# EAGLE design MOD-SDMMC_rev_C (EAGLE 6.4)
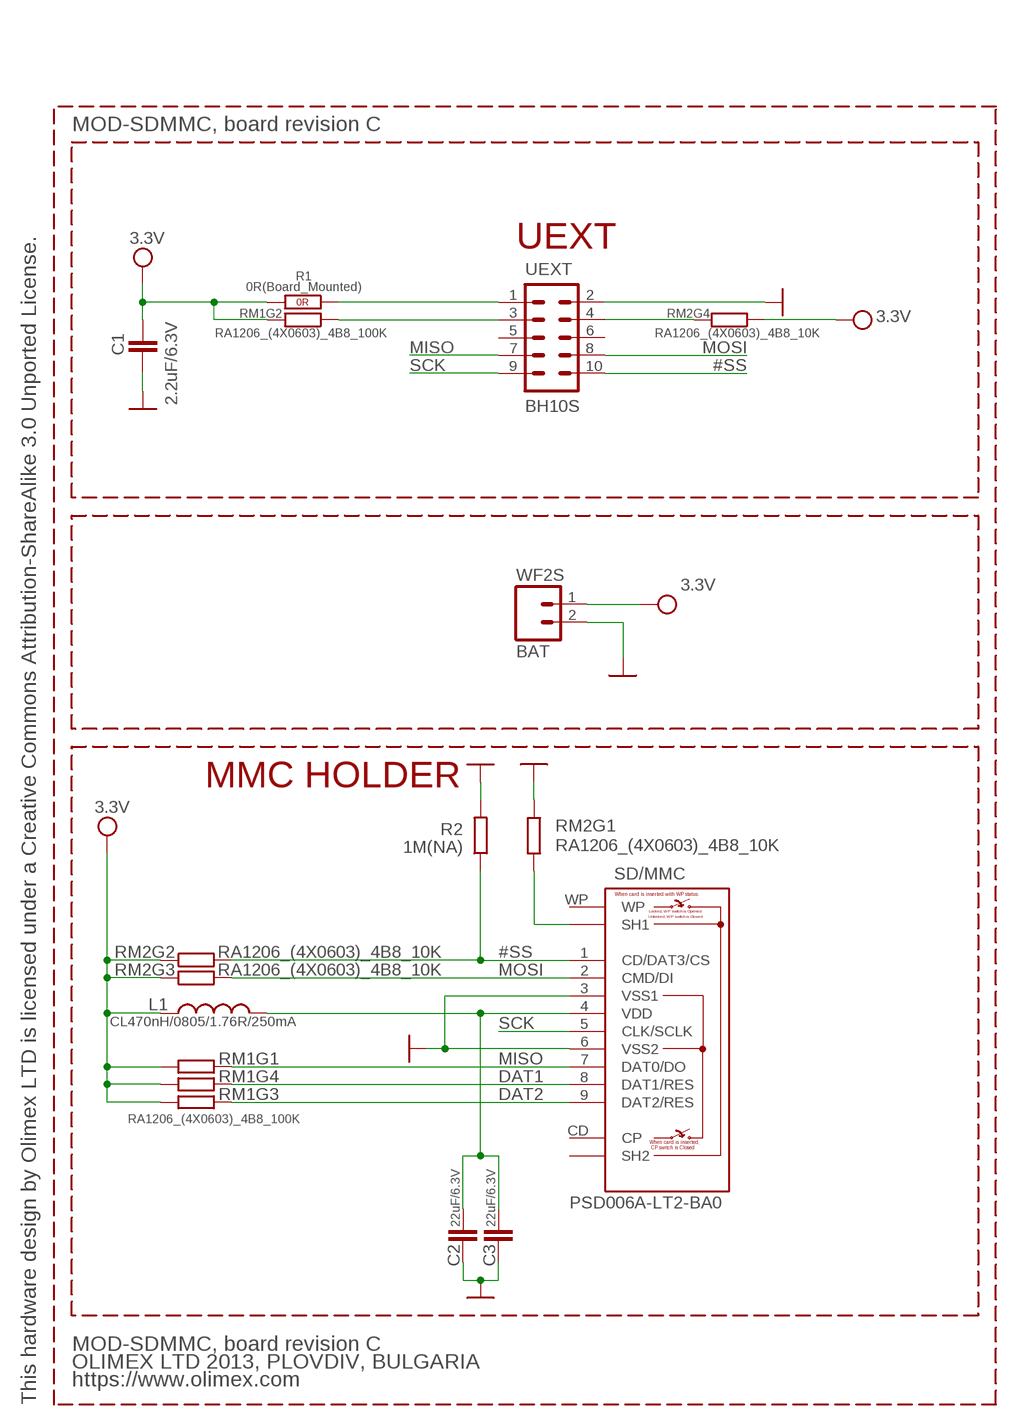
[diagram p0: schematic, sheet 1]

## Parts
BAT  WF2S  CON2PV2-2.54MM  [CON2.54MM-2-0]
C1  2.2uF/6.3V  C-EUC0603_DWS  [C0603_DWS]
C2  22uF/6.3V  C-EUC0603_DWS  [C0603_DWS]
C3  22uF/6.3V  C-EUC0603_DWS  [C0603_DWS]
L1  CL470nH/0805/1.76R/250mA  L-USL0805_5MIL_DWS  [L0805_5MIL_DWS]
R1  0R(Board_Mounted)  R_0R0R(NA)  [0603_0R]
R2  1M(NA)  R-EU_R0603_5MIL_DWS  [R0603_5MIL_DWS]
RM1  RA1206_(4X0603)_4B8_100K  R_MATRIX_4E  [R_MATRIX_4]
RM2  RA1206_(4X0603)_4B8_10K  R_MATRIX_4E  [R_MATRIX_4]
SD/MMC  PSD006A-LT2-BA0  SD_CARD_PSD006A-LT2-BA0  [SD_CARD]
UEXT  BH10S  ML10  [ML10-MALE]

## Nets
#SS: R2.1 RM2.2.2 SD/MMC.1(CD/DAT3/CS) UEXT.10
DAT1: RM1.4.1 SD/MMC.8(DAT1/RES)
DAT2: RM1.3.1 SD/MMC.9(DAT2/RES)
GND: BAT.2 C1.1 C2.1 C3.1 R2.2 RM2.1.1 SD/MMC.3(VSS1) SD/MMC.6(VSS2) UEXT.2
MISO: RM1.1.1 SD/MMC.7(DAT0/DO) UEXT.7
MOSI: RM2.3.2 SD/MMC.2(CMD/DI) UEXT.8
N$1: RM2.1.2 SD/MMC.SH1
N$2: RM1.2.1 UEXT.3
N$3 [PWR]: R1.1(1.1) UEXT.1
N$4: RM2.4.2 UEXT.4
SCK: SD/MMC.5(CLK/SCLK) UEXT.9
VCC [PWR]: BAT.1 C1.2 L1.1 R1.2(1.2) RM1.1.2 RM1.2.2 RM1.3.2 RM1.4.2 RM2.2.1 RM2.3.1 RM2.4.1 ; supply symbol labelled 3.3V
VDD_SD: C2.2 C3.2 L1.2 SD/MMC.4(VDD)
Unconnected: SD/MMC.CD(CP) SD/MMC.SH2 SD/MMC.WP UEXT.5 UEXT.6

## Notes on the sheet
- MOD-SDMMC, board revision C
- UEXT
- MMC HOLDER
- MOD-SDMMC, board revision C
- OLIMEX LTD 2013, PLOVDIV, BULGARIA
- https://www.olimex.com
- This hardware design by Olimex LTD is licensed under a Creative Commons Attribution-ShareAlike 3.0 Unported License.

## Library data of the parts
BAT = DOUBLE-SIDE:CON2: CONNECTORS - 2 PINS
C1-C3 = rcl:C-EU: CAPACITOR, European symbol
L1 = rcl:L-US: INDUCTOR, American symbol
R1 = OLIMEX_DISCRET:R_0R
R2 = rcl:R-EU_: RESISTOR, European symbol
RM1 RM2 = OLIMEX_DISCRET:R_MATRIX_4E
SD/MMC = OLIMEX_CONNECTORS:SD_CARD
UEXT = con-harting-ml:ML10: HARTING

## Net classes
0 default: width 0.107 mm
1 PWR: width 0.107 mm, drill 0.2 mm, clearance 0.076 mm

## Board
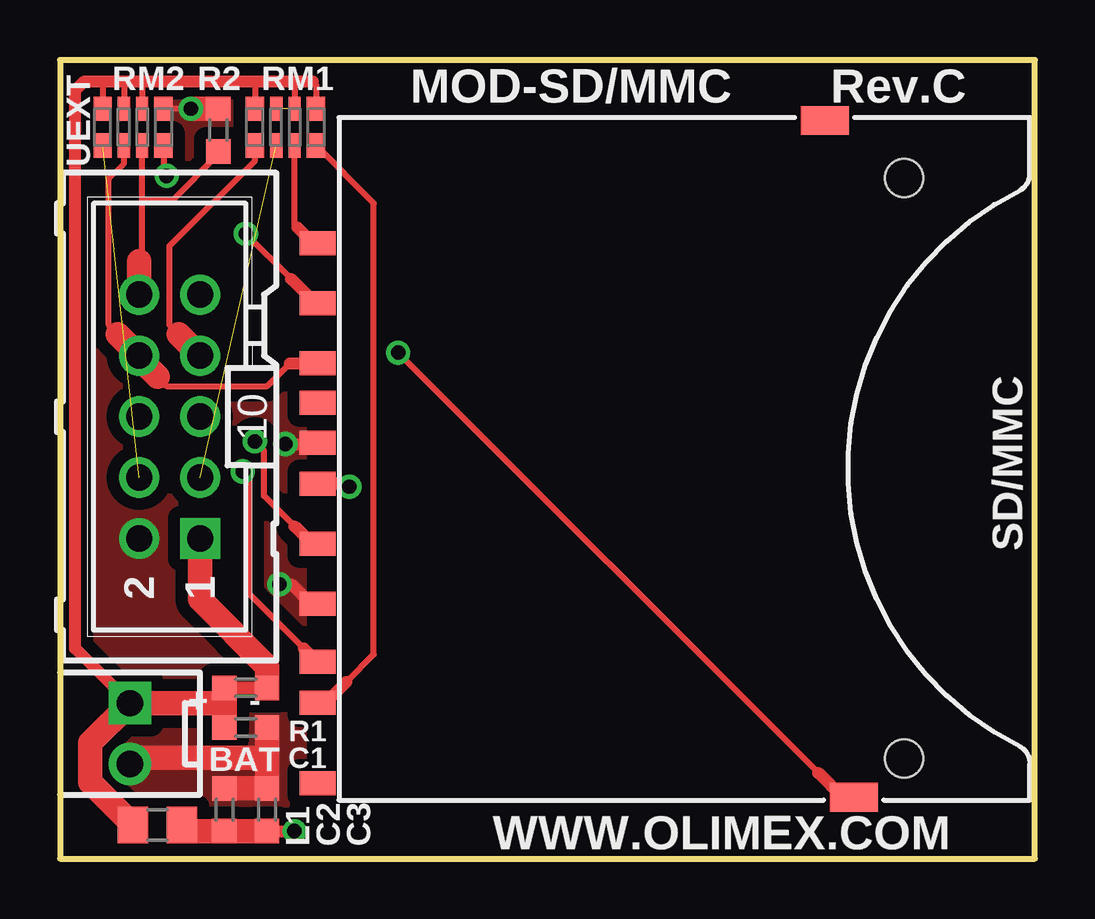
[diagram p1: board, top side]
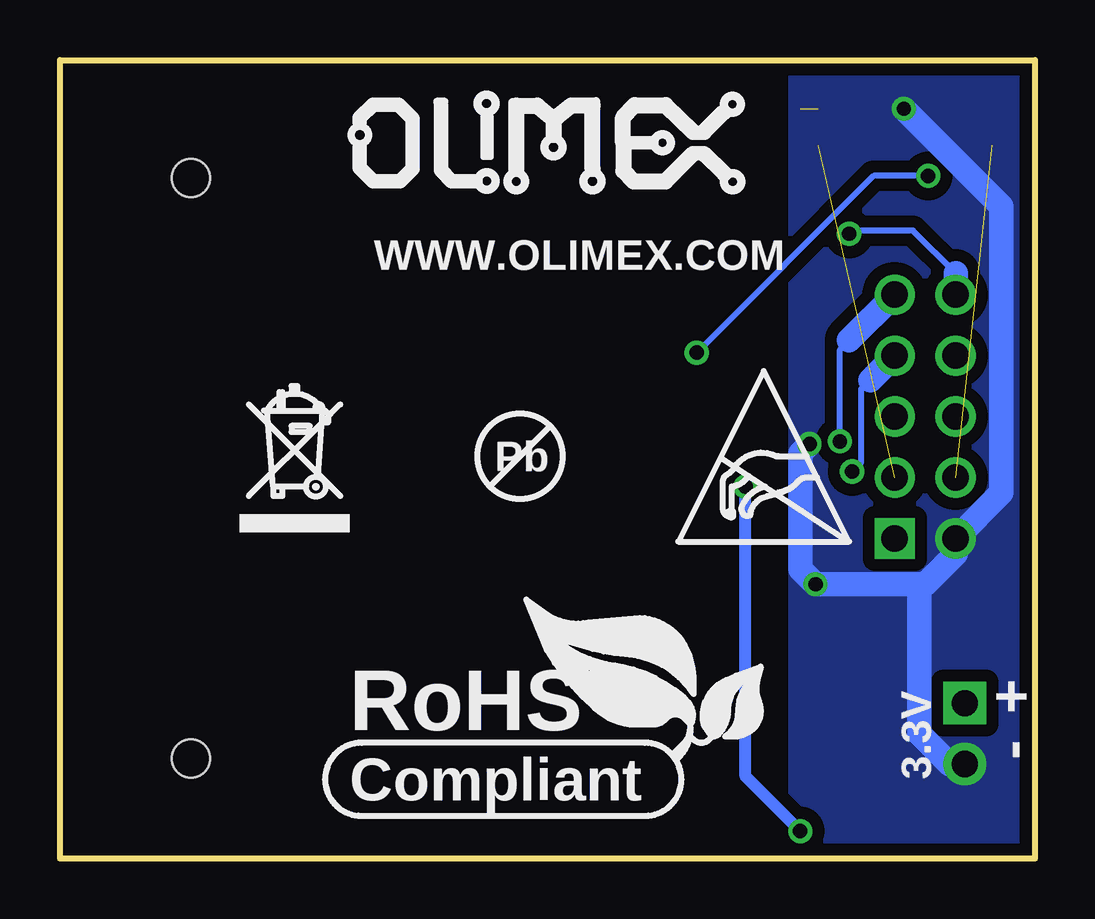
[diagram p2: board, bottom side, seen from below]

Size 40.64 x 33.27 mm. Coordinates in mm from the lower left corner, seen from the top.
Outline: 0,0 40.64,0 40.64,33.27 0,33.27 0,0
Copper layers (1+16): Top 0.035mm / dielectric 1.5mm / Bottom 0.035mm
Design rules "default": minimum track width 10mil, minimum drill 23mil, track to track 8mil, track to pad 8mil, pad to pad 8mil, via to via 8mil, smd to smd 1mil, copper to edge 10mil, drill to drill 8mil, minimum pad ring 10mil, minimum via ring 8mil, stop-mask expansion 4mil, vias tented up to drill 25mil, thermal gap 12mil

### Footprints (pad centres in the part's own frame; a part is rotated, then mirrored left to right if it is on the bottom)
CON2.54MM-2-0 = drill 1.092 pad 1.778 square: 1 -1.27,0 | drill 1.092 pad 1.778: 2 1.27,0
C0603_DWS = smd 1.016 x 1.016: 1 -0.889,0; 2 0.889,0
L0805_5MIL_DWS = smd 1.27 x 1.524: 1 -1.016,0; 2 1.016,0
0603_0R = smd 1.016 x 1.016: 1 -0.889,0; 2 0.889,0
R0603_5MIL_DWS = smd 1.016 x 1.016: 1 -0.889,0; 2 0.889,0
R_MATRIX_4 = smd 1.016 x 0.762: 1.1 -0.762,1.27; 1.2 0.762,1.27; 4.1 -0.762,-1.27; 4.2 0.762,-1.27 | smd 1.016 x 0.508: 2.1 -0.762,0.381; 2.2 0.762,0.381; 3.1 -0.762,-0.381; 3.2 0.762,-0.381
SD_CARD = smd 1 x 1.5: 1 6.88,15.3; 2 4.38,15.3; 3 1.08,15.3; 4 -0.63,15.3; 5 -3.13,15.3; 6 -5.63,15.3; 7 -8.06,15.3; 8 -9.76,15.3; 9 9.38,15.3; CD 2.73,15.3; WP -13.11,15.3 | smd 1.2 x 2: SH1 -13.7,-7.05; SH2 14.5,-5.85 | hole 1.6: -12.09,-9.15; 12.1,-9.15
ML10-MALE = drill 1.1 pad 1.676 square: 1 -5.08,-1.27 | drill 1.1 pad 1.676: 2 -5.08,1.27; 3 -2.54,-1.27; 4 -2.54,1.27; 5 0,-1.27; 6 0,1.27; 7 2.54,-1.27; 8 2.54,1.27; 9 5.08,-1.27; 10 5.08,1.27

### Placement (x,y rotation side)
BAT  2.92,5.21 270 top
C1  7.75,5.46 180 top
C2  6.86,2.03 270 top
C3  8.64,2.03 270 top
L1  4.06,1.4 0 top
R1  7.75,7.11 180 top
R2  6.6,30.35 90 top
RM1  9.4,30.48 90 top
RM2  3.05,30.48 270 top
SD/MMC  26.04,16.26 90 top
U$1  [PB_SMALL]  21.46,16.76 0 bottom
U$2  [RECYCLE_BIN1/8]  33.15,13.59 0 bottom
U$3  [ESD_SYMBOL]  14.86,13.21 0 bottom
U$4  [ROHS]  28.57,2.41 0 bottom
U$5  [OLIMEX1_V]  10.92,27.56 0 bottom
UEXT  4.57,18.41 90 top

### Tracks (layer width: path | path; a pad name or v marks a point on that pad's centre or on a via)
#SS  (via drill 0.6)
  Top 0.254: v7.75,26.04 9.63,24.15 | 3.3,24.89 3.43,25.02 3.43,27.43 | 3.43,27.43 RM2.2.2 | R2.1 6.6,29.34 4.7,27.43 3.43,27.43
  Top 0.508: 9.63,24.15 10.65,23.14 SD/MMC.1
  Top 1.016: UEXT.10 3.3,24.89
  Bottom 0.254: v7.75,26.04 7.62,26.16 5.08,26.16 3.3,24.38
  Bottom 1.016: UEXT.10 3.3,24.38
DAT1
  Top 0.254: 11.94,7.37 13.08,8.51 13.08,27.3 RM1.4.1
  Top 0.508: SD/MMC.8 11.07,6.5 11.94,7.37
DAT2
  Top 0.254: 9.91,26.29 9.78,26.42 RM1.3.1
  Top 0.508: SD/MMC.9 10.56,25.64 9.91,26.29
GND  (via drill 0.6)
  Top 0.254: v5.46,31.24 RM2.1.1
  Top 0.508: v9.4,17.27 10.67,17.27 SD/MMC.3 | v9.14,11.43 9.65,11.43 10.46,10.63 SD/MMC.6
  Top 1.016: C2.1 C3.1 8.64,4.19 | v5.46,31.24 R2.2 | UEXT.2 3.43,13.21 | BAT.2 3.17,4.19 8.64,4.19 | 8.64,4.19 C1.1
  Bottom 1.016: 4.83,11.43 v9.14,11.43 9.78,12.06 9.78,16.89 v9.4,17.27 | 4.83,11.43 4.57,11.43 3.3,12.7 UEXT.2 1.4,15.24 1.4,27.18 v5.46,31.24 | BAT.2 3.56,3.94 4.83,5.21 4.83,11.43
  pour Top (isolate 0.508, no thermals): -2.54,37.08 10.16,37.08 10.16,-2.54 -2.54,-2.54
  pour Bottom (isolate 0.508, no thermals): -5.08,-5.08 10.16,-5.08 10.16,39.62 -5.08,39.62
MISO  (via drill 0.6)
  Top 0.254: 4.95,21.84 4.57,22.23 4.57,25.53 8.13,29.08 RM1.1.1 | 10.16,8.76 7.87,11.05 7.87,15.88 v7.62,16.13
  Top 0.508: SD/MMC.7 10.16,8.76
  Top 1.016: UEXT.7 4.95,21.84
  Bottom 0.254: v7.62,16.13 7.24,16.51 7.24,19.56 6.86,19.94
  Bottom 1.016: 6.86,19.94 UEXT.7
MOSI
  Top 0.254: 4.06,20.07 4.45,19.68 8.64,19.68 9.59,20.64 | 2.41,21.84 2.03,22.23 2.03,28.32 2.67,28.96 RM2.3.2
  Top 0.508: 9.59,20.64 SD/MMC.2
  Top 1.016: 4.06,20.07 3.3,20.83 UEXT.8 2.41,21.84
N$1  (via drill 0.6)
  Top 0.254: v14.1,21.08 31.61,3.57 | RM2.1.2 4.32,28.57 v4.45,28.45
  Top 0.508: 31.61,3.57 32.62,2.56 SD/MMC.SH1
  Bottom 0.254: v4.45,28.45 6.73,28.45 v14.1,21.08
N$2  (1 unrouted)
N$3
  Top 1.016: UEXT.1 5.84,10.79 8.64,8 R1.1
N$4  (1 unrouted)
SCK  (via drill 0.6)
  Top 0.254: 9.78,13.84 8.51,15.11 8.51,17 v8.13,17.38
  Top 0.508: SD/MMC.5 10.5,13.13 9.78,13.84
  Bottom 0.254: v8.13,17.38 8.13,21.21 7.75,21.59
  Bottom 1.016: 7.75,21.59 UEXT.9
VCC  (1 unrouted)
  Top 0.254: RM1.4.2 10.67,32.26 10.54,32.38 | 1.78,32.38 RM2.4.1 | 3.43,32.38 RM2.2.1 | 2.67,32.38 RM2.3.1 | 8.13,32.38 RM1.1.2 | 9.78,32.38 RM1.3.2
  Top 0.508: BAT.1 0.64,8.76 0.64,32 1.02,32.38 1.78,32.38 2.67,32.38 3.43,32.38 8.13,32.38 9.02,32.38 9.78,32.38 10.54,32.38
  Top 1.016: L1.1 1.27,3.17 1.27,4.83 BAT.1 6.86,6.48 | 6.86,6.48 C1.2 | 6.86,6.48 R1.2
VDD_SD  (via drill 0.6)
  Top 0.508: C3.2 v9.78,1.14 | v12.06,15.49 11.93,15.63 SD/MMC.4
  Top 1.016: C3.2 C2.2 5.33,1.14 L1.2
  Bottom 0.508: v9.78,1.14 12.06,3.43 v12.06,15.49

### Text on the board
tNames: MOD-SD/MMC | Rev.C | + | - | WWW.OLIMEX.COM
bNames: WWW.OLIMEX.COM | + | - | 3.3V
